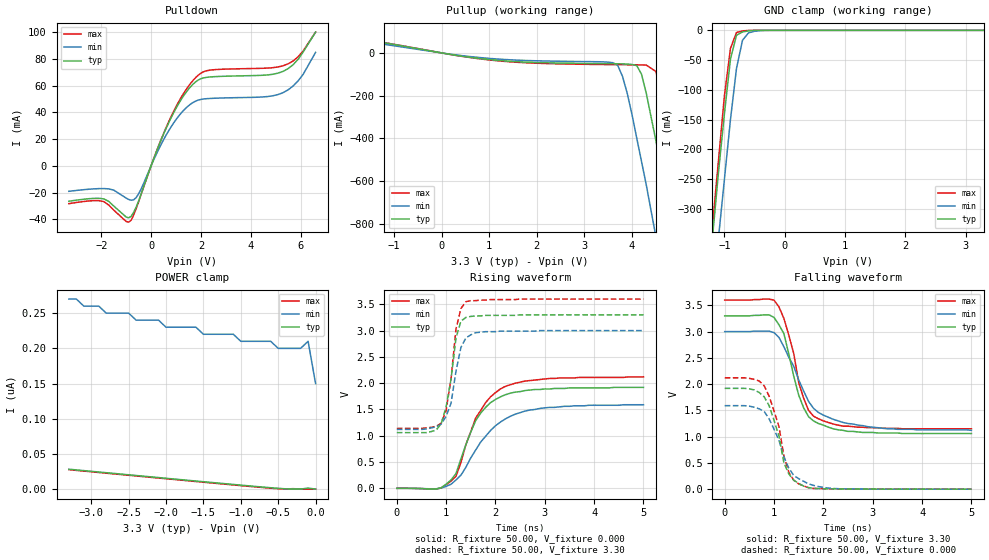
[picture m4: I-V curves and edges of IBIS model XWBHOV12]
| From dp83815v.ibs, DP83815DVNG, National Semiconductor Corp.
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|   Model XWBHOV12
[Model]   XWBHOV12
Model_type   I/O
Polarity   Non-Inverting
Enable   Active-High
Vinl =   0.80V
Vinh =   2.00V
Vmeas =   1.50V
Cref =  20.00pF
Rref = 100.00k
C_comp   5.00pF   5.00pF   5.00pF
[Temperature Range]   25.00   0.14k   0.000
[Voltage Range]   3.30V   3.00V   3.60V
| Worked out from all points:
|   slope of the pulldown table from 0 to 0.495 V, typ, clamps not added: 21.1 ohm
|   slope of the pullup table from 0 to 0.495 V, typ, clamps not added: 28 ohm
|   GND clamp passes 1 mA (typ) near -0.60 V on its own axis
|   rising waveform, R_fixture 50.00, V_fixture 0.000: 20-80 % time 559ps typ, 775ps min, 585ps max; typ from 0 V to 1.92 V
|   rising waveform, R_fixture 50.00, V_fixture 3.30: 20-80 % time 212ps typ, 237ps min, 195ps max; typ from 1.06 V to 3.3 V
|   falling waveform, R_fixture 50.00, V_fixture 3.30: 20-80 % time 397ps typ, 612ps min, 395ps max; typ from 3.3 V to 1.06 V
|   falling waveform, R_fixture 50.00, V_fixture 0.000: 20-80 % time 336ps typ, 424ps min, 340ps max; typ from 1.92 V to 0 V
[Pulldown]
| voltage   I(typ)   I(min)   I(max)
-3.3V     -26.48mA   -19.06mA   -28.28mA
-1.9V     -24.72mA   -17mA      -26.74mA
-900mV    -38.88mA   -25.16mA   -42.15mA
-700mV    -34.77mA   -25.46mA   -36.84mA
-500mV    -26.29mA   -20.89mA   -26.78mA
700mV     31.96mA    26.07mA    32.67mA
1.3V      52.23mA    41.38mA    54.01mA
1.8V      62.95mA    48.5mA     66.19mA
2.4V      66.48mA    50.41mA    71.64mA
5.3V      70.67mA    54.75mA    74.83mA
5.9V      79.7mA     63.55mA    81.56mA
6.6V      100mA      84.82mA    100mA
[Pullup]
| voltage   I(typ)   I(min)   I(max)
-3.3V     110mA      27.63mA    110mA
-2.7V     96.2mA     77.72mA    99.58mA
1V        -31.19mA   -25.59mA   -32.8mA
3.6V      -50.7mA    -46.04mA   -54.92mA
3.9V      -52.21mA   -190mA     -55.51mA
4.1V      -59.85mA   -400mA     -55.87mA
4.3V      -190mA     -620mA     -57.12mA
4.5V      -410mA     -860mA     -86.87mA
4.9V      -880mA     -1.34A     -500mA
5.1V      -1.13A     -1.58A     -740mA
5.3V      -1.37A     -1.82A     -990mA
6.6V      -2.99A     -3.43A     -2.6A
[GND_clamp]
| voltage   I(typ)   I(min)   I(max)
-3.3V     -2.93A     -3.01A     -2.91A
-1.2V     -350mA     -460mA     -330mA
-1.1V     -240mA     -350mA     -220mA
-1V       -140mA     -250mA     -110mA
-900mV    -48.33mA   -150mA     -30.32mA
-800mV    -8.29mA    -63.99mA   -3.67mA
-700mV    -2.68mA    -16.62mA   -950uA
-600mV    -980uA     -4.2mA     -170uA
-500mV    -190uA     -1.55mA    -15.48uA
-200mV    -43.2nA    -10.78uA   -890pA
3.3V      110pA      200nA      36.28pA
[POWER_clamp]
| voltage   I(typ)   I(min)   I(max)
-3.3V     28.37nA    270nA      27.7nA
-2.8V     23.41nA    250nA      22.74nA
-2V       15.5nA     230nA      14.84nA
-1.6V     11.58nA    230nA      10.91nA
-1.5V     10.6nA     220nA      9.93nA
-1.1V     6.72nA     220nA      6.05nA
-1V       5.77nA     210nA      5.1nA
-600mV    2.06nA     210nA      1.43nA
-500mV    1.22nA     200nA      640pA
-200mV    130pA      200nA      130pA
-100mV    1.59nA     210nA      43.62pA
0V        110pA      150nA      39.7pA
[Ramp]
| variable   typ   min   max
dV/dt_r   1.88/0.28n   1.69/0.37n   2.06/0.28n
dV/dt_f   1.90/0.29n   1.72/0.41n   2.08/0.28n
R_load = 0.50k
[Rising Waveform]
R_fixture = 50.00
V_fixture = 0.000
V_fixture_min = 0.000
V_fixture_max = 0.000
| time   V(typ)   V(min)   V(max)
0s        91.7uV     80.5uV     100uV
800ps     -12.13mV   -8.34mV    -14.39mV
1.1ns     160mV      77.84mV    140mV
1.2ns     280mV      160mV      230mV
1.3ns     560mV      250mV      490mV
1.6ns     1.29V      730mV      1.34V
1.9ns     1.63V      1.1V       1.74V
2.2ns     1.78V      1.32V      1.94V
3.1ns     1.89V      1.54V      2.09V
5ns       1.92V      1.59V      2.12V
[Rising Waveform]
R_fixture = 50.00
V_fixture = 3.30
V_fixture_min = 3.00
V_fixture_max = 3.60
| time   V(typ)   V(min)   V(max)
0s        1.06V      1.12V      1.14V
600ps     1.06V      1.13V      1.15V
900ps     1.23V      1.22V      1.24V
1ns       1.55V      1.37V      1.48V
1.1ns     2.08V      1.62V      2.09V
1.2ns     2.86V      2.23V      3.03V
1.3ns     3.18V      2.68V      3.42V
1.4ns     3.25V      2.86V      3.55V
1.8ns     3.29V      2.98V      3.58V
5ns       3.3V       3V         3.6V
[Falling Waveform]
R_fixture = 50.00
V_fixture = 3.30
V_fixture_min = 3.00
V_fixture_max = 3.60
| time   V(typ)   V(min)   V(max)
0s        3.3V       3V         3.6V
1ns       3.27V      2.98V      3.6V
1.2ns     2.96V      2.71V      3.25V
1.4ns     2.15V      2.34V      2.58V
1.5ns     1.79V      2.08V      2.03V
1.6ns     1.55V      1.87V      1.73V
1.7ns     1.38V      1.67V      1.5V
1.9ns     1.25V      1.46V      1.34V
2.9ns     1.08V      1.19V      1.17V
5ns       1.06V      1.12V      1.15V
[Falling Waveform]
R_fixture = 50.00
V_fixture = 0.000
V_fixture_min = 0.000
V_fixture_max = 0.000
| time   V(typ)   V(min)   V(max)
0s        1.92V      1.59V      2.12V
500ps     1.91V      1.58V      2.11V
800ps     1.76V      1.48V      1.97V
900ps     1.59V      1.34V      1.77V
1.1ns     1.01V      930mV      1.19V
1.2ns     500mV      610mV      630mV
1.3ns     290mV      400mV      320mV
1.5ns     110mV      200mV      100mV
2.2ns     5.46mV     13.38mV    5.12mV
5ns       120uV      160uV      150uV
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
